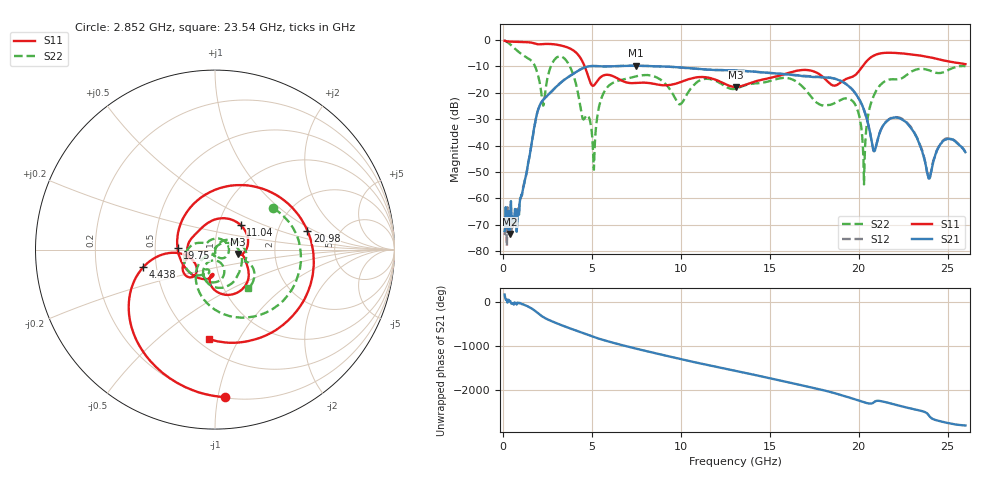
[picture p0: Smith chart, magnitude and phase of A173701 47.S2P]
!  2-Port S-parameters saved by WinCal
! VAR MeasName=S-Parameters (CALIBRATED_DATA) read from VNA (N5245A)
! VAR MeasDate=2017-6-7 10:31:32
! VAR NAME=A173701 47
! VAR FILENAME=A173701 47.S2P
! VAR DATE=2017-6-7 10:31:32
! VAR PHYS_PORTS=1,2
# Hz S DB R 50
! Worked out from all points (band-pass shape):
!   801 points, 100 MHz to 26 GHz, reference 50 ohm
!   highest |S21| = -9.80 dB at 7.481 GHz (marker M1); lowest = -73.5 dB at 391.4 MHz (marker M2)
!   |S21| within 3 dB of the highest: 3.978 GHz to 15.48 GHz (11.5 GHz wide, 118 % of centre)
!   lowest |S11| = -17.8 dB at 13.11 GHz (marker M3), VSWR 1.29, Z = 64.3 - j3.14 ohm
!   |S11| at or under -10 dB: 4.598 GHz to 20.22 GHz (15.62 GHz wide, 126 % of centre)
!   |S22| runs from -54.7 to -0.2 dB; largest |S21 - S12| = 0.005
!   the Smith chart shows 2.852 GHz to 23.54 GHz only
!   S11 on the Smith chart (normalised r, x): 2.852 GHz: 0.21, -1.05; 4.438 GHz: 0.42, -0.10; 11.04 GHz: 1.28, +0.36; 19.75 GHz: 0.65, +0.01; 20.98 GHz: 2.94, +0.86; 23.54 GHz: 0.57, -0.76
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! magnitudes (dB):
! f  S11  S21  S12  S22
! 100 MHz  -0.3  -72.3  -73.9  -0.2
! 391.4 MHz  -0.7  -73.5  -70.3  -1.6
! 909.4 MHz  -0.8  -66.2  -65.7  -4.7
! 2.269 GHz  -1.6  -22.7  -22.7  -24.9
! 2.852 GHz  -1.7  -18.8  -18.7  -8.0
! 4.438 GHz  -7.7  -10.9  -10.9  -28.6
! 5.118 GHz  -17.2  -9.9  -9.9  -49.1
! 5.766 GHz  -13.3  -10.1  -10.1  -18.9
! 7.481 GHz  -16.3  -9.8  -9.8  -13.8
! 8.744 GHz  -17.0  -10.0  -10.0  -14.6
! 11.04 GHz  -14.1  -11.0  -11.1  -15.4
! 13.05 GHz  -17.8  -11.6  -11.6  -18.5
! 13.11 GHz  -17.8  -11.6  -11.6  -18.4
! 17.39 GHz  -11.7  -14.0  -13.9  -22.0
! 19.75 GHz  -13.6  -19.6  -19.7  -23.9
! 20.3 GHz  -9.3  -26.5  -26.7  -54.7
! 20.98 GHz  -5.6  -40.1  -40.1  -19.3
! 21.69 GHz  -4.9  -30.2  -30.1  -15.1
! 23.54 GHz  -6.0  -41.7  -41.4  -11.0
! 23.96 GHz  -6.5  -52.5  -52.3  -11.5
! 24.83 GHz  -7.9  -37.9  -37.6  -12.1
! 26 GHz  -9.2  -42.5  -42.2  -10.0
